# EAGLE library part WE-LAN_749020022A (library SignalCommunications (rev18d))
WE-LAN LAN Transformer Characteristics Compliant with standards: IEEE 802.3u, IEEE 802.3ab, IEEE 802.3af, IEEE 802.3at and upcoming IEE 802.3bt SMD Applications Ethernet speed up to 10 Gbit/s Power over Ethernet PoE and PoE+ Compliant with most IC’s for Ethernet applications such as Intel, AMD, Microchip and Realtek Hub, Router, Switches, IPcameras, IoT Details see: http://katalog.we-online.de/en/pbs/WE-LAN/749020022A? 2016 (C) Würth Elektronik
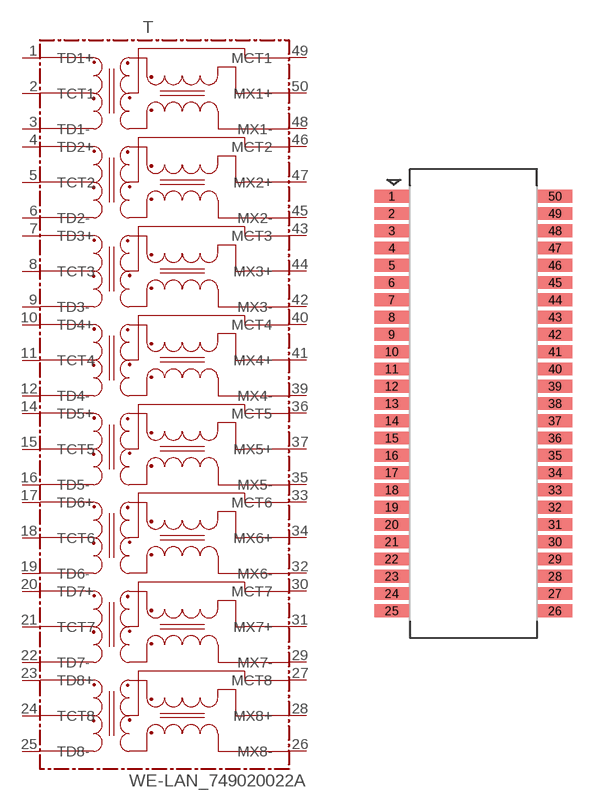
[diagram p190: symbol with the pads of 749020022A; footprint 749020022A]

Designator prefix T

## WE-LAN_749020022A  [749020022A]
1  TD1+
2  TCT1
3  TD1-
4  TD2+
5  TCT2
6  TD2-
7  TD3+
8  TCT3
9  TD3-
10  TD4+
11  TCT4
12  TD4-
14  TD5+
15  TCT5
16  TD5-
17  TD6+
18  TCT6
19  TD6-
20  TD7+
21  TCT7
22  TD7-
23  TD8+
24  TCT8
25  TD8-
26  MX8-
27  MCT8
28  MX8+
29  MX7-
30  MCT7
31  MX7+
32  MX6-
33  MCT6
34  MX6+
35  MX5-
36  MCT5
37  MX5+
39  MX4-
40  MCT4
41  MX4+
42  MX3-
43  MCT3
44  MX3+
45  MX2-
46  MCT2
47  MX2+
48  MX1-
49  MCT1
50  MX1+

## Footprint 749020022A (pad centres in mm)
smd 2.03 x 0.76: 1 -4.825,12.24; 2 -4.825,11.22; 3 -4.825,10.2; 4 -4.825,9.18; 5 -4.825,8.16; 6 -4.825,7.14; 7 -4.825,6.12; 8 -4.825,5.1; 9 -4.825,4.08; 10 -4.825,3.06; 11 -4.825,2.04; 12 -4.825,1.02; 13 -4.825,0; 14 -4.825,-1.02; 15 -4.825,-2.04; 16 -4.825,-3.06; 17 -4.825,-4.08; 18 -4.825,-5.1; 19 -4.825,-6.12; 20 -4.825,-7.14; 21 -4.825,-8.16; 22 -4.825,-9.18; 23 -4.825,-10.2; 24 -4.825,-11.22; 25 -4.825,-12.24; 26 4.825,-12.24; 27 4.825,-11.22; 28 4.825,-10.2; 29 4.825,-9.18; 30 4.825,-8.16; 31 4.825,-7.14; 32 4.825,-6.12; 33 4.825,-5.1; 34 4.825,-4.08; 35 4.825,-3.06; 36 4.825,-2.04; 37 4.825,-1.02; 38 4.825,0; 39 4.825,1.02; 40 4.825,2.04; 41 4.825,3.06; 42 4.825,4.08; 43 4.825,5.1; 44 4.825,6.12; 45 4.825,7.14; 46 4.825,8.16; 47 4.825,9.18; 48 4.825,10.2; 49 4.825,11.22; 50 4.825,12.24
